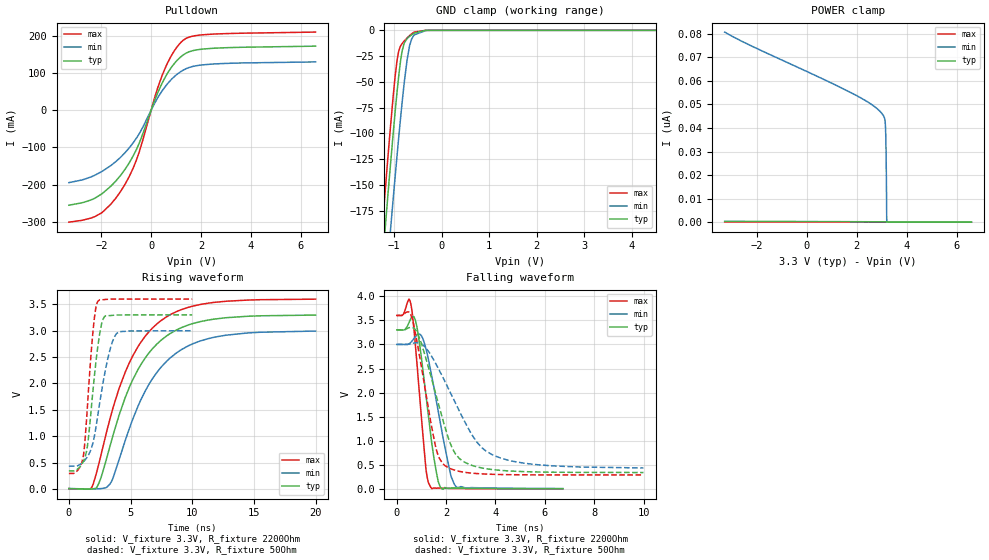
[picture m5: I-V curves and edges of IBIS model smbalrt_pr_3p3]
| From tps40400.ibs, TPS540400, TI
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|   smbalrt_pr_3p3 Model
[Model]   smbalrt_pr_3p3
Model_type   Open_sink
Polarity   Inverting
Vmeas = 1.65
Vref = 3.3
Cref = 2pF
Rref = 2200
|   typ   min   max
|   (nom PVT)   (fast PVT)   (slow PVT)
C_comp   1.150e-12   1.129e-12   1.173e-12
| Where nom  PVT is Nominal Process, 3.3V, 25C
|   Fast PVT is Strong Process,  3.4V, -40C
|   Slow PVT is Weak Process,   3.2V, 125C
[Voltage Range]   3.3   3.2   3.4
|Junction Temperature
[Temperature Range]   25   125   -40
[Pullup Reference]   3.3   3.2   3.4
[Pulldown Reference]   0   0   0
[Power Clamp Reference]   3.3   3.2   3.4
[GND Clamp Reference]   0   0   0
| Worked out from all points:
|   slope of the pulldown table from 0 to 0.495 V, typ, clamps not added: 6.2 ohm
|   GND clamp passes 1 mA (typ) near -0.42 V on its own axis
|   falling waveform, V_fixture 3.3V, R_fixture 2200Ohm: 20-80 % time 481ps typ, 660ps min, 356ps max; typ from 3.3 V to 0.008 V
|   rising waveform, V_fixture 3.3V, R_fixture 2200Ohm: 20-80 % time 3.54ns typ, 3.69ns min, 3.46ns max; typ from 0.008 V to 3.3 V
|   falling waveform, V_fixture 3.3V, R_fixture 50Ohm: 20-80 % time 998ps typ, 1.59ns min, 682ps max; typ from 3.3 V to 0.344 V
|   rising waveform, V_fixture 3.3V, R_fixture 50Ohm: 20-80 % time 782ps typ, 1.15ns min, 617ps max; typ from 0.344 V to 3.3 V
[Pulldown]
|   Voltage   I(typ)   I(min)   I(max)
-3.3V     -255.3mA   -194.7mA   -301.1mA
-2.41V    -241.1mA   -179.3mA   -289.8mA
-2.001V   -225.9mA   -165.7mA   -276.5mA
-1.221V   -174.9mA   -126.2mA   -218mA
-861.6mV  -139.6mA   -99.81mA   -175.9mA
-576.8mV  -103.8mA   -73.77mA   -131.6mA
148.5mV   27.58mA    19.62mA    35.46mA
460.4mV   75.5mA     53.98mA    96.63mA
858mV     119.4mA    85.93mA    152.1mA
1.293V    149mA      108mA      188.4mA
2.422V    166.3mA    124mA      204.5mA
6.597V    172.3mA    129.9mA    210.1mA
[GND Clamp]
|   Voltage   I(typ)   I(min)   I(max)
-3.3V     -1.486A    -1.512A    -1.478A
-1.277V   -244.6mA   -306.4mA   -209.5mA
-1.127V   -159.8mA   -223.3mA   -123.2mA
-1.092V   -140.4mA   -204mA     -103.6mA
-1.019V   -101.2mA   -164.7mA   -65.03mA
-940.4mV  -62.25mA   -124.1mA   -30.94mA
-903mV    -45.55mA   -105.3mA   -20.73mA
-828.3mV  -20.01mA   -69.82mA   -12.85mA
-724mV    -8.058mA   -28.57mA   -7.408mA
-672.8mV  -5.897mA   -15.15mA   -5.152mA
-570.4mV  -2.564mA   -4.36mA    -1.648mA
6.597V    0A         0A         0A
[POWER Clamp]
|   Voltage   I(typ)   I(min)   I(max)
-3.3V     396.6pA    80.72nA    94.42pA
1.782V    213.1pA    54.91nA    23.02pA
2.504V    185.7pA    50.61nA    12.87pA
2.998V    163.7pA    46.27nA    5.93pA
3.116V    156.8pA    43.98nA    4.264pA
3.148V    154.5pA    40.78nA    3.813pA
3.161V    153.5pA    36.79nA    3.633pA
3.174V    152.5pA    29.42nA    3.452pA
3.186V    151.4pA    17.72nA    3.272pA
3.199V    150.2pA    1.198nA    3.091pA
3.206V    149.5pA    0A         3.001pA
6.597V    0A         0A         0A
[Ramp]
R_load = 2200
|   typ   min   max
dV/dt_r   1.97358/3.5421e-09   1.79048/3.68195e-09   2.15508/3.4539e-09
dV/dt_f   1.97543/4.80974e-10   1.79406/6.60576e-10   2.15613/3.56033e-10
[Falling Waveform]
V_fixture = 3.3V
V_fixture_min = 3V
V_fixture_max = 3.6V
R_fixture = 2200Ohm
|   Time   V(typ)   V(min)   V(max)
0s        3.3V       3V         3.6V
494ps     3.451V     3.012V     3.94V
570ps     3.536V     3.042V     3.842V
810ps     3.377V     3.196V     2.652V
1.182ns   1.949V     2.909V     413.8mV
1.414ns   964.9mV    2.349V     14.89mV
1.76ns    46.56mV    1.388V     21.53mV
2.198ns   22.69mV    267.2mV    14.9mV
2.4ns     22.47mV    52.94mV    13mV
6.73ns    7.934mV    11.86mV    6.481mV
[Rising Waveform]
V_fixture = 3.3V
V_fixture_min = 3V
V_fixture_max = 3.6V
R_fixture = 2200Ohm
|   Time   V(typ)   V(min)   V(max)
0s        7.622mV    9.764mV    6.455mV
1.862ns   410.9uV    1.224mV    32.04mV
2.446ns   116.9mV    5.554mV    492.4mV
3.326ns   805.3mV    93.41mV    1.323V
4.096ns   1.417V     575.9mV    1.921V
5.19ns    2.076V     1.33V      2.527V
7.404ns   2.805V     2.289V     3.18V
9.118ns   3.058V     2.641V     3.399V
11.34ns   3.204V     2.853V     3.524V
20ns      3.297V     2.994V     3.598V
[Falling Waveform]
V_fixture = 3.3V
V_fixture_min = 3V
V_fixture_max = 3.6V
R_fixture = 50Ohm
|   Time   V(typ)   V(min)   V(max)
0s        3.3V       3V         3.6V
606ps     3.353V     3.019V     3.567V
922ps     3.128V     3.026V     2.763V
1.58ns    1.972V     2.6V       861.8mV
1.94ns    1.308V     2.243V     492.5mV
2.256ns   837.9mV    1.912V     408.3mV
2.556ns   626.5mV    1.598V     366.4mV
3.246ns   461.8mV    974.4mV    322.6mV
3.928ns   402.3mV    699.4mV    306.3mV
9.998ns   344.3mV    438.8mV    294mV
[Rising Waveform]
V_fixture = 3.3V
V_fixture_min = 3V
V_fixture_max = 3.6V
R_fixture = 50Ohm
|   Time   V(typ)   V(min)   V(max)
0s        344mV      433.3mV    294mV
756ps     387.5mV    444.8mV    365.1mV
1.18ns    523.4mV    518mV      628.7mV
1.504ns   812.5mV    612.4mV    1.559V
1.946ns   1.846V     867.4mV    2.963V
2.334ns   2.678V     1.38V      3.552V
2.884ns   3.264V     2.161V     3.59V
3.428ns   3.289V     2.717V     3.599V
3.866ns   3.297V     2.948V     3.6V
9.998ns   3.3V       3V         3.6V
